(* Logix 5000 AddOnInstructionDefinition export AMCI_ANG1E_Program_Motor_Current; software revision 20.03 *)

ADD_ON_INSTRUCTION AMCI_ANG1E_Program_Motor_Current   (* revision 1.1, vendor AMCI *)
// Revision note:
// Version 1.1 added the slot_axis number and the input parameters can now be tags or discrete values.
VAR_INPUT
   slot_axis_number : INT; {required}
   motor_current : INT;
END_VAR
VAR_IN_OUT
   AMCI_ANG1E_output_data : INT[10]; {required}
END_VAR
VAR
   command_data_block : INT[10];
        [0]   // Command Bits MSW
        [1]   // Command Bits LSW
        [2]   // Upper Target Position
        [3]   // Lower Target Position
        [4]   // Upper Programmed Speed
        [5]   // Lower Programmed Speed
   index : INT;
END_VAR

ROUTINE Logic   (* ladder *)
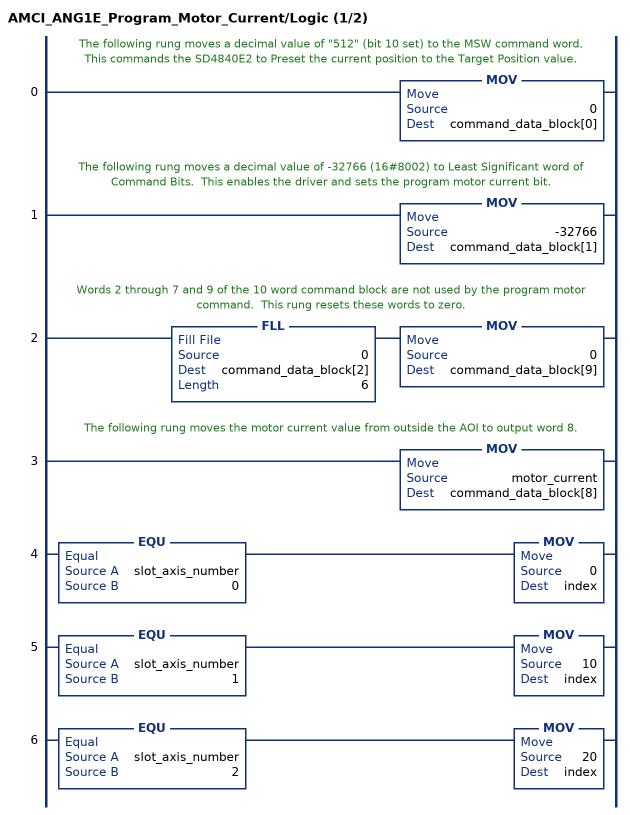
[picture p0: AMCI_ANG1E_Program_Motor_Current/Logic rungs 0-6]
   // The following rung moves a decimal value of "512" (bit 10 set) to the MSW command word.  This commands the SD4840E2 to Preset the current position to the Target Position value.
   0: MOV(0,command_data_block[0]);
   // The following rung moves a decimal value of -32766 (16#8002) to Least Significant word of Command Bits.  This enables the driver and sets the program motor current bit.
   1: MOV(-32766,command_data_block[1]);
   // Words 2 through 7 and 9 of the 10 word command block are not used by the program motor command.  This rung resets these words to zero.
   2: FLL(0,command_data_block[2],6)MOV(0,command_data_block[9]);
   // The following rung moves the motor current value from outside the AOI to output word 8.
   3: MOV(motor_current,command_data_block[8]);
   4: EQU(slot_axis_number,0)MOV(0,index);
   5: EQU(slot_axis_number,1)MOV(10,index);
   6: EQU(slot_axis_number,2)MOV(20,index);
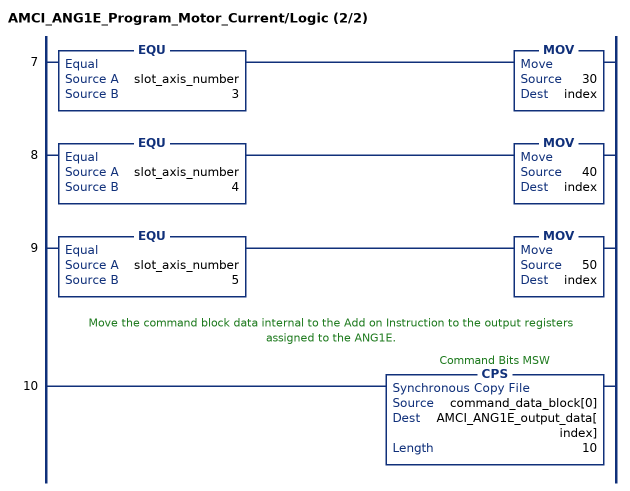
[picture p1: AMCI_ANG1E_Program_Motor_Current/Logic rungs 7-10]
   7: EQU(slot_axis_number,3)MOV(30,index);
   8: EQU(slot_axis_number,4)MOV(40,index);
   9: EQU(slot_axis_number,5)MOV(50,index);
   // Move the command block data internal to the Add on Instruction to the output registers assigned to the ANG1E.
   10: CPS(command_data_block[0],AMCI_ANG1E_output_data[index],10);
END_ROUTINE
END_ADD_ON_INSTRUCTION
